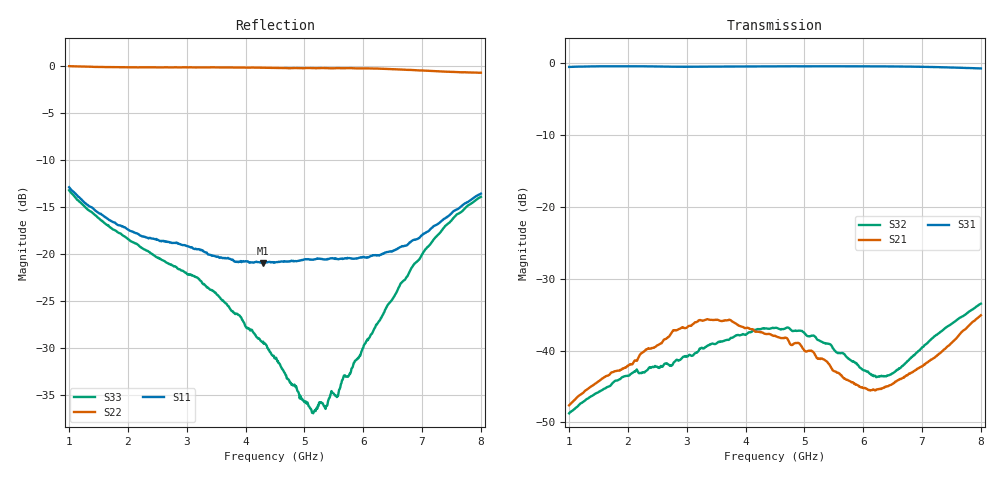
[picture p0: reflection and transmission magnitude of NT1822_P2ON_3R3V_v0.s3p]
! NT1822 PC-P2 ON state
! Port1:PC, Port2:P1, Port3:P2
! VDD=3.3V, VCTL=1.2V
# hz S ma R 50
! 3 Port Network Data from SP1.SP block
! freq  magS11  angS11  magS12  angS12  magS13  angS13
!  magS21  angS21
!  magS22  angS22  magS23  angS23
!  magS31  angS31  magS32  angS32
!  magS33  angS33
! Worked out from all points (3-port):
!   701 points, 1 GHz to 8 GHz, reference 50 ohm
!   strongest paths, dB at 1 GHz, 2.75 GHz, 4.5 GHz, 6.25 GHz, 8 GHz:
!     S31: -0.6, -0.5, -0.5, -0.5, -0.8
!     S21: -47.6, -37.4, -37.9, -45.4, -35.1
!     S32: -48.7, -42.0, -36.9, -43.6, -33.5
!   lowest |S11| = -21.0 dB at 4.3 GHz (marker M1), VSWR 1.20, Z = 54.8 - j8.12 ohm
!   |S11| at or under -10 dB: start of sweep to end of sweep
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1e9  0.2266 -77.1  0.004189 79.0  0.9362 1.8
     0.004163 78.9  1.002 -13.0  0.003662 73.4
     0.9357 1.6  0.003662 73.4  0.2184 -77.3
2.04e9  0.1327 -77.6  0.008038 80.6  0.9471 -14.2
        0.008051 80.2  0.9877 -25.6  0.00683 70.4
        0.9465 -14.4  0.006841 70.1  0.1172 -91.3
3.21e9  0.1058 -64.4  0.0163 65.5  0.9387 -26.6
        0.01624 65.4  0.9864 -38.7  0.01015 75.8
        0.9384 -27.0  0.01012 75.4  0.07344 -102.8
4.3e9  0.08956 -55.2  0.01326 41.3  0.9431 -37.5
       0.01324 41.3  0.9823 -52.1  0.01426 60.7
       0.9425 -37.8  0.0143 60.7  0.03404 -126.2
4.5e9  0.09 -55.7  0.01266 39.9  0.9438 -39.6
       0.01269 39.9  0.98 -54.9  0.01435 56.3
       0.9432 -40.0  0.01437 56.0  0.02791 -129.1
5.13e9  0.09306 -62.7  0.009933 36.0  0.9449 -45.9
        0.009874 36.5  0.9779 -64.5  0.01267 45.4
        0.9447 -46.4  0.01267 44.9  0.01421 -114.1
5.36e9  0.09339 -67.9  0.008499 37.5  0.9452 -48.3
        0.008497 37.7  0.9787 -68.4  0.0112 43.9
        0.9454 -48.8  0.01116 43.0  0.01491 -107.6
5.96e9  0.09598 -88.3  0.005573 61.7  0.9446 -54.4
        0.005554 62.0  0.9761 -79.9  0.007511 52.5
        0.9443 -55.1  0.007517 52.0  0.02943 -116.2
6.39e9  0.1019 -107.3  0.005649 90.7  0.943 -59.2
        0.005636 90.3  0.9695 -88.4  0.006617 81.2
        0.9429 -59.5  0.006612 81.1  0.05162 -124.7
8e9  0.2095 -172.9  0.01764 136.9  0.9134 -76.7
     0.01758 136.8  0.9244 -119.7  0.02117 119.9
     0.9133 -77.2  0.02117 119.5  0.2014 -137.2
